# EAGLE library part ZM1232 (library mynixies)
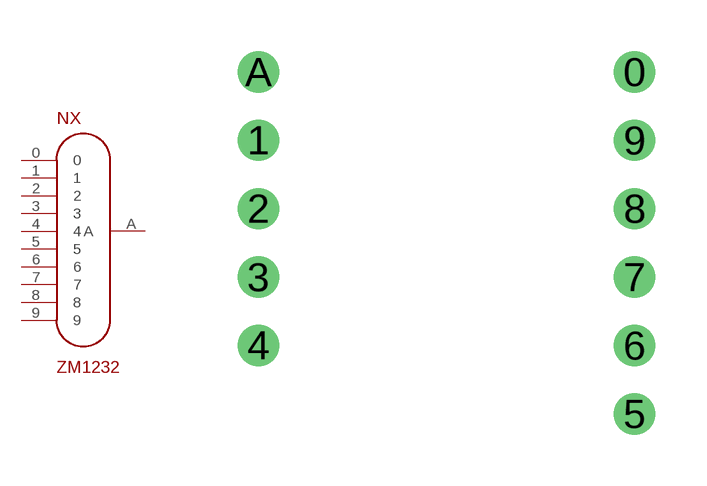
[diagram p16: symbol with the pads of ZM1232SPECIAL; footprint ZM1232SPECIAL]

Designator prefix NX

## ZM1232SPECIAL  [ZM1232SPECIAL]
0  0  pas
1  1  pas
2  2  pas
3  3  pas
4  4  pas
5  5  pas
6  6  pas
7  7  pas
8  8  pas
9  9  pas
A  A  pas

## Footprint ZM1232SPECIAL (pad centres in mm)
drill 0.7: 0 5.5,5; 1 -5.5,3; 2 -5.5,1; 3 -5.5,-1; 4 -5.5,-3; 5 5.5,-5; 6 5.5,-3; 7 5.5,-1; 8 5.5,1; 9 5.5,3; A -5.5,5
